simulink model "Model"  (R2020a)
settings: Solver=ode15s  StartTime=0.0  StopTime=tsim  FixedStep=0.1  MaxStep=1  RelTol=1e-5
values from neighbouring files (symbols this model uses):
  C = Fc*cpc/(Fh*cph)    [calcblock.m]    (also in calcblock2.m; calcblock3.m; eNTU.m = m.c*cp.c/(m.h*cp.h); Main.m = [zeros(1,2*N-1),1])
  d_tstep = 300    [Main.m]    (also in Main_OL.m = 3000; runTestCalcBlk.m; runTransf.m = [500; 50000; 70000; 130000; 50000; 50000]; runTransfOL.m = [500 5000 7000 13000])
  dFh = 0;0.2*Fh    [Main.m]    (also in runTransf.m = 2; runTransfOL.m = 0)
  dTcin = 2    [Main.m]    (also in runTransf.m = 0; runTransfOL.m = 0)
  dThin = 0;2    [Main.m]    (also in runTransf.m = 0; runTransfOL.m = 0)
  dThsp = 0    [Main.m]    (also in Main_OL.m = Thsp0*[0.01;-0.01]; runTestCalcBlk.m = 1)
  Fc0 = 5    [Main.m]    (also in Main_OL.m; runTestCalcBlk.m; runTransf.m; runTransfOL.m)
  Fh = d(1)    [calcblock.m]    (also in calcblock2.m; calcblock3.m; HEXode.m; Main.m = 3)
  KI = 0    [Main.m]    (also in Main_OL.m = 1; runTransf.m = 1/kS(i)*1/tauCS(i); runTransfOL.m = 1/kS(i)*1/tauCS(i))
  Kp = 1/kv*tauv/(tauC+thetav)    [Main.m]    (also in Main_OL.m = 0; runTransf.m = 1)
  nd = size(d0,2)    [Main.m]    (also in Main_OL.m; runTestCalcBlk.m; runTransf.m = size(d0,1); runTransfOL.m)
  np = size(p,2)    [Main.m]    (also in Main_OL.m; runTestCalcBlk.m; runH2Psim.m = length(param); runTransf.m)
  nu = 1    [Main.m]    (also in Main_OL.m; runTestCalcBlk.m; runH2Psim.m = length(u0); runTransf.m)
  nx = size(x0,1)    [Main.m]    (also in Main_OL.m; runTestCalcBlk.m; H2P_Turbine_driven.m = param(end); runTD.m = length(x0))
  p = [N, Fc0, rhoc, rhoh,U,A,cpc,cph]    [Main.m]    (also in Main_OL.m; runTestCalcBlk.m; NonlinearMap.m = [U;A;Fc(i);Fh;cpc;cph;Tcin;Thin]; runTransf.m = [N, Fc0, rhoc, rhoh, U0, A,cpc,cph])
  pi_ff = 0    [Main.m]    (also in Main_OL.m; runTransfOL.m)
  tau = 10    [Main.m]    (also in Main_OL.m = 130; runTransf.m = [100;310;400]; runTransfOL.m = [100;310;400])
  Tcin = d(2)    [calcblock.m]    (also in calcblock2.m; calcblock3.m; HEXode.m; Main.m = 293.15)
  theta = 0    [Main.m]    (also in Main_OL.m = 40; runTransf.m = [40;60;60]; runTransfOL.m = [40;60;60]; BaseCase.m)
  Thin = d(3)    [calcblock.m]    (also in calcblock2.m; calcblock3.m; HEXode.m; Main.m = 343.15)
  Thsp = Thsp0+dThsp    [Main.m]    (also in Main_OL.m = sp(j); runTestCalcBlk.m; runTransf.m = Thsp0; runTransfOL.m = Thsp0)
  Thsp0 = Thend(end)    [Main.m]    (also in Main_OL.m; runTestCalcBlk.m; runTransf.m = x0(end-1);  2.971202611676064e+02; runTransfOL.m = x0(end);  2.971202611676064e+02)
  tstep = 100    [Main.m]    (also in Main_OL.m = 500; runTransf.m = 10000; runTransfOL.m)
  v0 = Tout.h    [Main.m]    (also in Main_OL.m = 1; runTD.m = v(end,:); runBD.m = v(end,:); runFP.m = v(end,:))
  vf = v0    [Main.m]    (also in runTransfOL.m = v00; runTransf.m = 0)
  x0 = [Tcend(1:N)'; Thend(1:N)']    [Main.m]    (also in Main_OL.m; runTestCalcBlk.m; runTD.m = [TE0;TD0;TSh0;MD0; MSh0;w0;TA0;0;0;0;0;0;0;0;0;0]; runBD.m = [TE0;TD0;TSh0;MD0; MSh0;w0;TA0;0;0;0;0;0;0;0;0;0])
undefined symbols (not defined in the file or in its folder): calcblock, HEXode

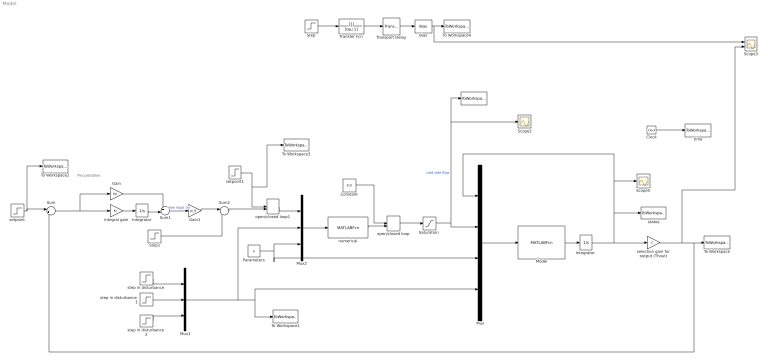
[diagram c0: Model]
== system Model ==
  note: PI-controller
  " " : ToWorkspace  VariableName=uc  SampleTime=-1
  Bias : Bias  Bias=24.44+273.15
  Clock : Clock
  Constant : Constant  Value=Fc0
  Gain : Gain  Gain=Kp
  Gain1 : Gain  Gain=pi_ff  Multiplication=Matrix(K*u)
  Integrator : Integrator
  "Integrator " : Integrator  InitialCondition=x0
  Model : MATLABFcn  MATLABFcn=HEXode(u(1:nx),u(nx+1:nx+nu),u(nx+nu+1:nx+nu+np),u(nx+nu+np+1:nx+nu+np+nd))  OutputDimensions=nx  Output1D=off
  Mux : Mux
  Mux1 : Mux  Inputs=3
  Mux2 : Mux  Inputs=3
  Parameters : Constant  Value=p
  "Saturation " : Saturate  UpperLimit=inf  LowerLimit=0
  Scope2 : Scope
  Scope3 : Scope  NumInputPorts=2
  Scope5 : Scope
  Step : Step  Time=tstep  After=dThsp  SampleTime=0
  Step1 : Step  Time=tstep  Before=v0  After=vf  SampleTime=0
  Sum : Sum  Inputs=|+-
  Sum1 : Sum  Inputs=++|
  Sum2 : Sum  Inputs=|++
  To Workspace : ToWorkspace  VariableName=Thout  SampleTime=-1
  To Workspace1 : ToWorkspace  VariableName=dsim  SampleTime=-1
  To Workspace2 : ToWorkspace  VariableName=Tsp  SampleTime=-1
  To Workspace3 : ToWorkspace  VariableName=ysp  SampleTime=-1
  To Workspace4 : ToWorkspace  VariableName=ytf  SampleTime=-1
  Transfer Fcn : TransferFcn  Denominator=[tau 1]
  Transport Delay : TransportDelay  DelayTime=theta
  integral gain : Gain  Gain=KI  Multiplication=Matrix(K*u)
  numerical : MATLABFcn  MATLABFcn=calcblock(u(nu),u(nu+1:nu+nd),u(nu+nd+1:nu+nd+np))
  open/closed loop : ManualSwitch  CurrentSetting=0
  open/closed loop1 : ManualSwitch  CurrentSetting=0
  selection gain for output (Thout) : Gain  Gain=C  Multiplication=Matrix(K*u)
  setpoint : Step  Time=tstep  Before=Thsp0  After=Thsp  SampleTime=0
  setpoint1 : Step  Time=tstep  Before=Thsp0  After=Thsp  SampleTime=0
  states : ToWorkspace  VariableName=T  SampleTime=-1
  step in disturbance : Step  Time=d_tstep(1)  Before=Fh  After=Fh+dFh  SampleTime=0
  step in disturbance1 : Step  Time=d_tstep(2)  Before=Tcin  After=Tcin+dTcin  SampleTime=0
  step in disturbance2 : Step  Time=d_tstep(3)  Before=Thin  After=Thin+dThin  SampleTime=0
  time : ToWorkspace  VariableName=t  SampleTime=-1
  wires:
  Model/1 -> "Integrator "/1
  "Integrator "/1 -> selection gain for output (Thout)/1, states/1, Mux/1, Scope5/1
  Mux/1 -> Model/1
  Clock/1 -> time/1
  Parameters/1 -> Mux/3, Mux2/3
  "Saturation "/1 -> Mux/2, Scope2/1, " "/1  "cold side flow"
  numerical/1 -> open/closed loop/2
  setpoint/1 -> To Workspace2/1, Sum/1
  Sum/1 -> Gain/1, integral gain/1
  integral gain/1 -> Integrator/1
  Sum1/1 -> Gain1/1  "new input (v)"
  selection gain for output (Thout)/1 -> Sum/2, To Workspace/1, Scope3/2
  Mux2/1 -> numerical/1
  Step1/1 -> Sum2/2
  open/closed loop/1 -> "Saturation "/1
  Constant/1 -> open/closed loop/1
  Integrator/1 -> Sum1/2
  open/closed loop1/1 -> Mux2/1
  setpoint1/1 -> To Workspace3/1, open/closed loop1/1
  Gain/1 -> Sum1/1
  Gain1/1 -> Sum2/1
  Sum2/1 -> open/closed loop1/2
  Bias/1 -> Scope3/1, To Workspace4/1
  Transport Delay/1 -> Bias/1
  Transfer Fcn/1 -> Transport Delay/1
  Step/1 -> Transfer Fcn/1
  Mux1/1 -> To Workspace1/1, Mux/4, Mux2/2
  step in disturbance/1 -> Mux1/1
  step in disturbance1/1 -> Mux1/2
  step in disturbance2/1 -> Mux1/3
